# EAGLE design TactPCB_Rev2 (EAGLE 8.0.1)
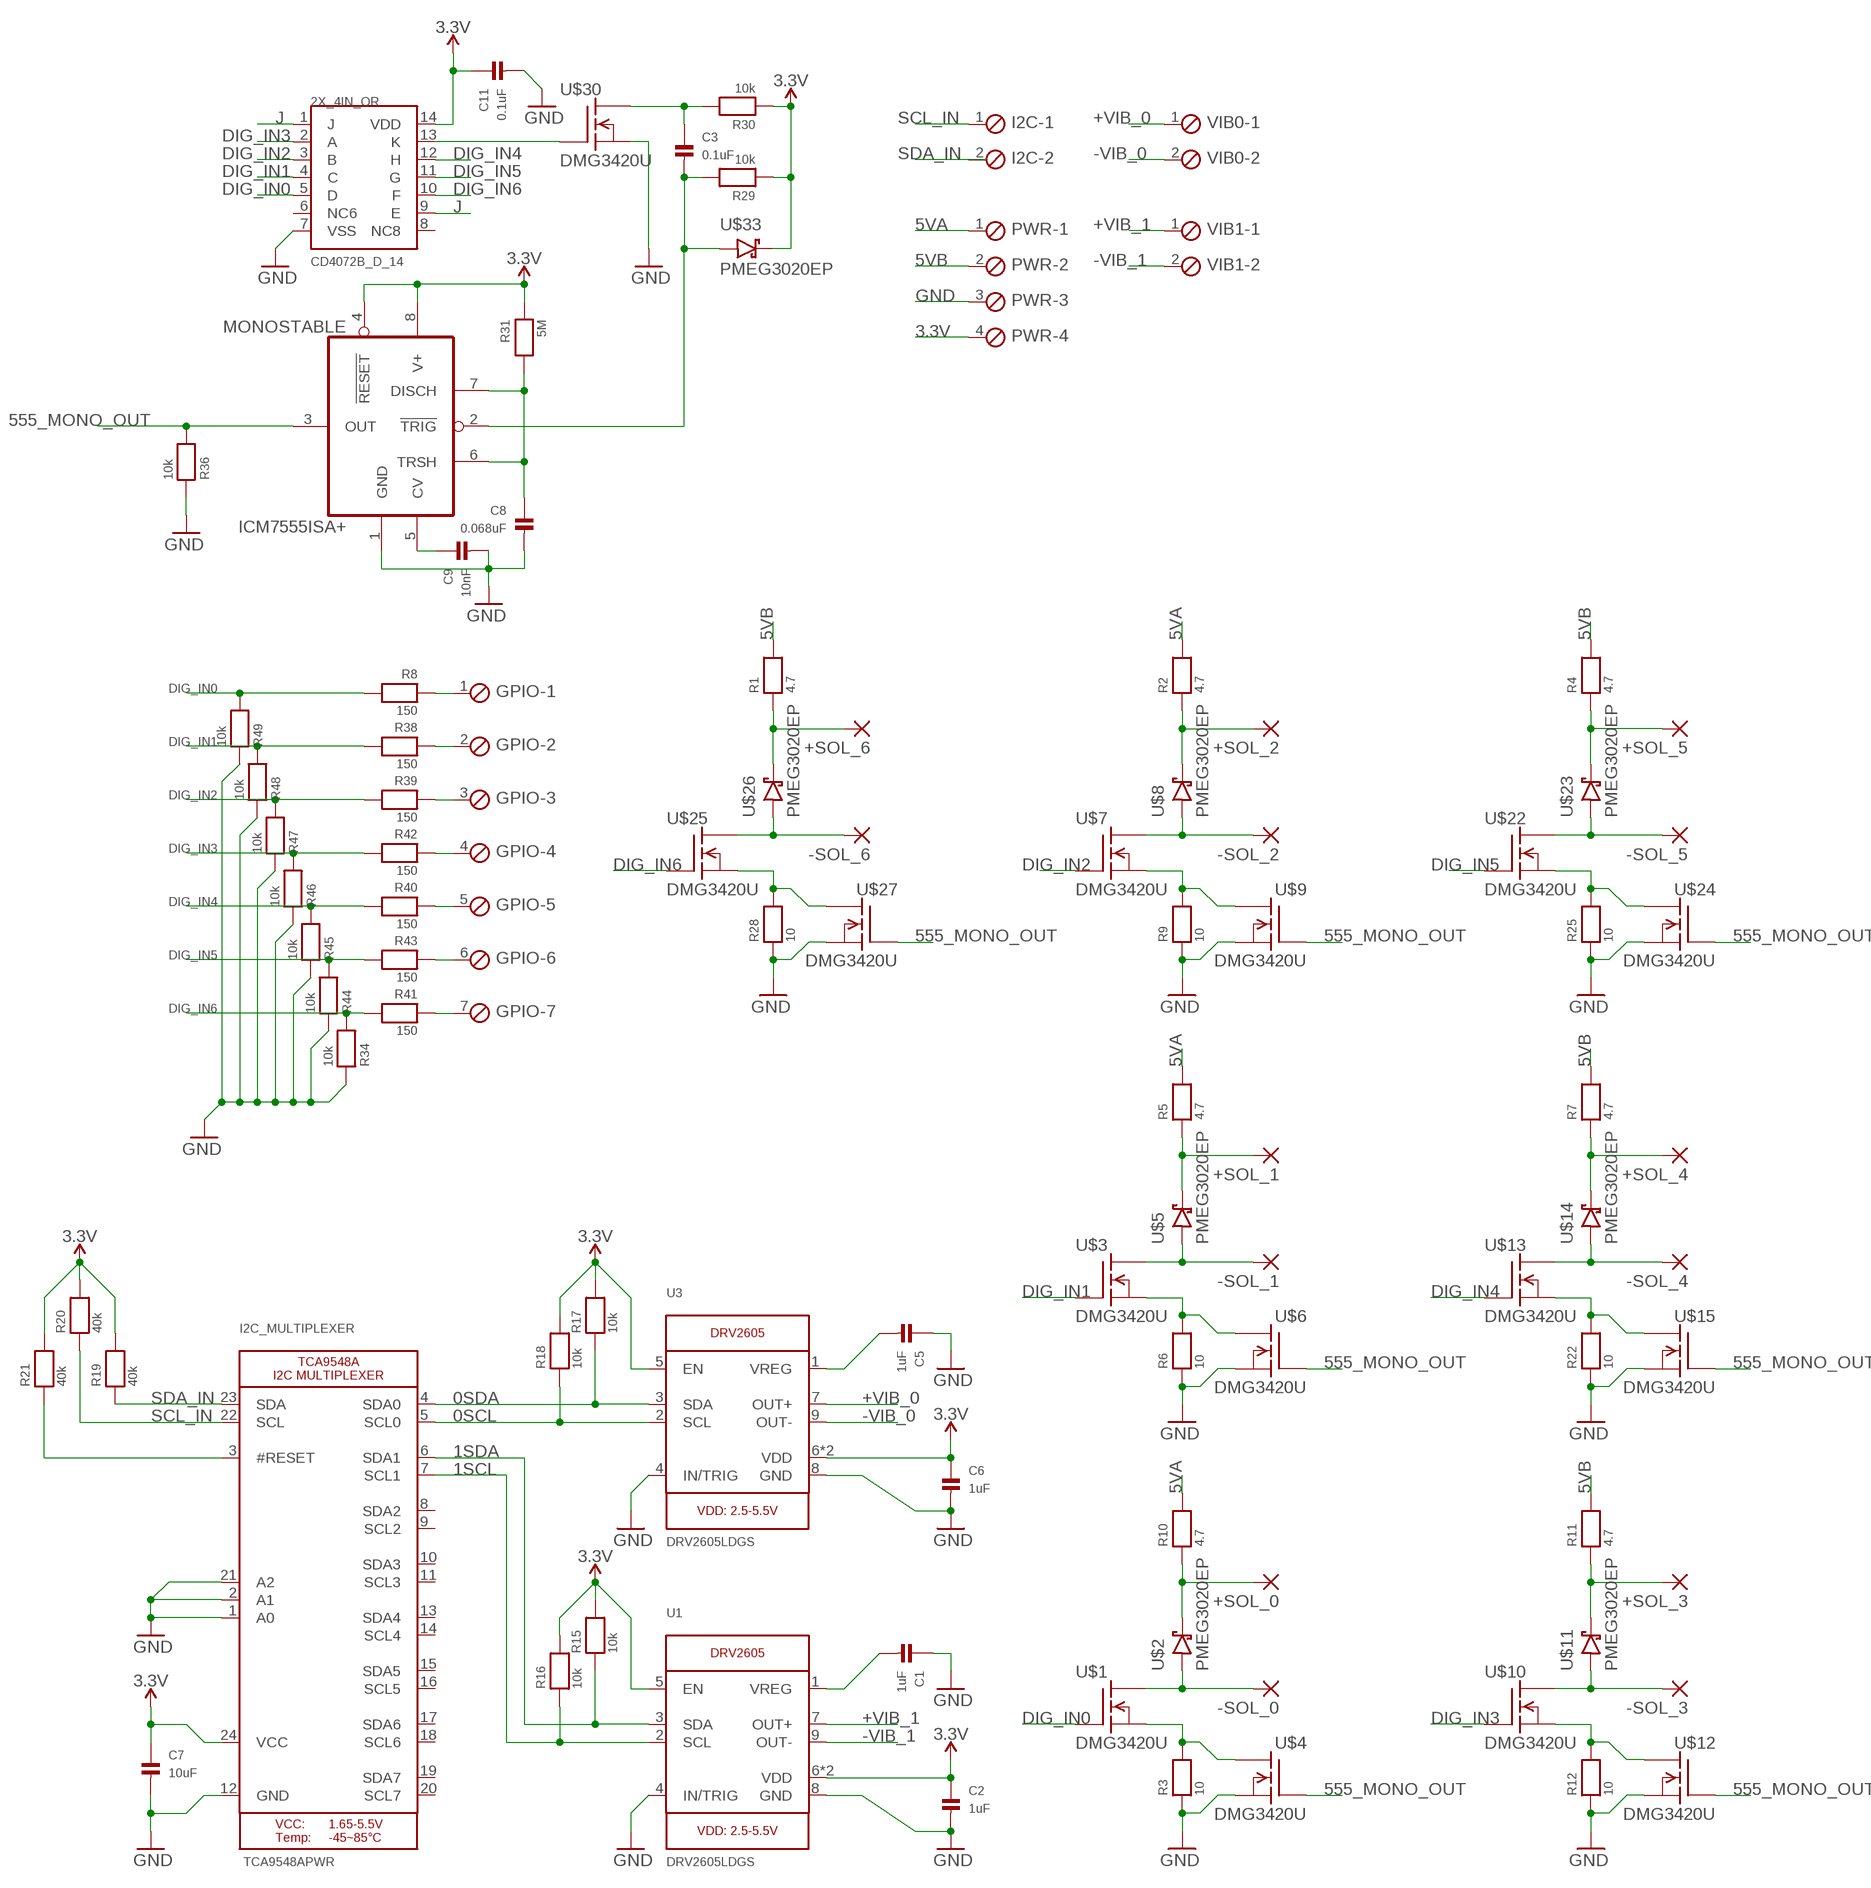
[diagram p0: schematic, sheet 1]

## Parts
2X_4IN_OR  CD4072B_D_14  [SOIC-14]
+SOL_0  2,15/1,0  [2,15/1,0]
+SOL_1  2,15/1,0  [2,15/1,0]
+SOL_2  2,15/1,0  [2,15/1,0]
+SOL_3  2,15/1,0  [2,15/1,0]
+SOL_4  2,15/1,0  [2,15/1,0]
+SOL_5  2,15/1,0  [2,15/1,0]
+SOL_6  2,15/1,0  [2,15/1,0]
-SOL_0  2,15/1,0  [2,15/1,0]
-SOL_1  2,15/1,0  [2,15/1,0]
-SOL_2  2,15/1,0  [2,15/1,0]
-SOL_3  2,15/1,0  [2,15/1,0]
-SOL_4  2,15/1,0  [2,15/1,0]
-SOL_5  2,15/1,0  [2,15/1,0]
-SOL_6  2,15/1,0  [2,15/1,0]
C1  1uF  CAP_CERAMIC0805  [0805]
C2  1uF  CAP_CERAMIC0805  [0805]
C3  0.1uF  CAP_CERAMIC0805  [0805]
C5  1uF  CAP_CERAMIC0805  [0805]
C6  1uF  CAP_CERAMIC0805  [0805]
C7  10uF  CAP_CERAMIC0805  [0805]
C8  0.068uF  CAP_CERAMIC0805  [0805]
C9  10nF  CAP_CERAMIC0805  [0805]
C11  0.1uF  CAP_CERAMIC0805  [0805]
GPIO  MPT7  [7POL254]
I2C  MPT2  [2POL254]
I2C_MULTIPLEXER  TCA9548APWR  TCA9548A  [TSSOP24]
MONOSTABLE  ICM7555ISA+  [SOIC-8]
PWR  MPT4  [4POL254]
R1  4.7  RESISTOR0805  [0805]
R2  4.7  RESISTOR0805  [0805]
R3  10  RESISTOR0805  [0805]
R4  4.7  RESISTOR0805  [0805]
R5  4.7  RESISTOR0805  [0805]
R6  10  RESISTOR0805  [0805]
R7  4.7  RESISTOR0805  [0805]
R8  150  RESISTOR0805  [0805]
R9  10  RESISTOR0805  [0805]
R10  4.7  RESISTOR0805  [0805]
R11  4.7  RESISTOR0805  [0805]
R12  10  RESISTOR0805  [0805]
R15  10k  RESISTOR0805  [0805]
R16  10k  RESISTOR0805  [0805]
R17  10k  RESISTOR0805  [0805]
R18  10k  RESISTOR0805  [0805]
R19  40k  RESISTOR0805  [0805]
R20  40k  RESISTOR0805  [0805]
R21  40k  RESISTOR0805  [0805]
R22  10  RESISTOR0805  [0805]
R25  10  RESISTOR0805  [0805]
R28  10  RESISTOR0805  [0805]
R29  10k  RESISTOR0805  [0805]
R30  10k  RESISTOR0805  [0805]
R31  5M  RESISTOR0805  [0805]
R34  10k  RESISTOR0805  [0805]
R36  10k  RESISTOR0805  [0805]
R38  150  RESISTOR0805  [0805]
R39  150  RESISTOR0805  [0805]
R40  150  RESISTOR0805  [0805]
R41  150  RESISTOR0805  [0805]
R42  150  RESISTOR0805  [0805]
R43  150  RESISTOR0805  [0805]
R44  10k  RESISTOR0805  [0805]
R45  10k  RESISTOR0805  [0805]
R46  10k  RESISTOR0805  [0805]
R47  10k  RESISTOR0805  [0805]
R48  10k  RESISTOR0805  [0805]
R49  10k  RESISTOR0805  [0805]
U1  DRV2605LDGS  DRV2605_SOP  [PSOP10]
U3  DRV2605LDGS  DRV2605_SOP  [PSOP10]
U$1  DMG3420U  [SOT23-3]
U$2  PMEG3020EP  [SOD128]
U$3  DMG3420U  [SOT23-3]
U$4  DMG3420U  [SOT23-3]
U$5  PMEG3020EP  [SOD128]
U$6  DMG3420U  [SOT23-3]
U$7  DMG3420U  [SOT23-3]
U$8  PMEG3020EP  [SOD128]
U$9  DMG3420U  [SOT23-3]
U$10  DMG3420U  [SOT23-3]
U$11  PMEG3020EP  [SOD128]
U$12  DMG3420U  [SOT23-3]
U$13  DMG3420U  [SOT23-3]
U$14  PMEG3020EP  [SOD128]
U$15  DMG3420U  [SOT23-3]
U$22  DMG3420U  [SOT23-3]
U$23  PMEG3020EP  [SOD128]
U$24  DMG3420U  [SOT23-3]
U$25  DMG3420U  [SOT23-3]
U$26  PMEG3020EP  [SOD128]
U$27  DMG3420U  [SOT23-3]
U$30  DMG3420U  [SOT23-3]
U$33  PMEG3020EP  [SOD128]
VIB0  MPT2  [2POL254]
VIB1  MPT2  [2POL254]

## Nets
0SCL: I2C_MULTIPLEXER.5(SCL0) R18.1 U3.2(SCL)
0SDA: I2C_MULTIPLEXER.4(SDA0) R17.1 U3.3(SDA)
1SCL: I2C_MULTIPLEXER.7(SCL1) R16.1 U1.2(SCL)
1SDA: I2C_MULTIPLEXER.6(SDA1) R15.1 U1.3(SDA)
3.3V: 2X_4IN_OR.14(VDD) C2.1 C6.1 C7.1 C11.1 I2C_MULTIPLEXER.24(VCC) MONOSTABLE.4(!RESET) MONOSTABLE.8(V+) PWR.4 R15.2 R16.2 R17.2 R18.2 R19.2 R20.2 R21.2 R29.1 R30.1 R31.1 U1.5(EN) U1.6(VDD) U1.10(VDD) U3.5(EN) U3.6(VDD) U3.10(VDD) U$33.2
5VA: PWR.1 R2.2 R5.2 R10.2
5VB: PWR.2 R1.2 R4.2 R7.2 R11.2
555_MONO_OUT: MONOSTABLE.3(OUT) R36.2 U$4.1(G) U$6.1(G) U$9.1(G) U$12.1(G) U$15.1(G) U$24.1(G) U$27.1(G)
+VIB_0: U3.7(OUT+) VIB0.1
+VIB_1: U1.7(OUT+) VIB1.1
-VIB_0: U3.9(OUT-) VIB0.2
-VIB_1: U1.9(OUT-) VIB1.2
DIG_IN0: 2X_4IN_OR.5(D) R8.2 R49.2 U$1.1(G)
DIG_IN1: 2X_4IN_OR.4(C) R38.2 R48.2 U$3.1(G)
DIG_IN2: 2X_4IN_OR.3(B) R39.2 R47.2 U$7.1(G)
DIG_IN3: 2X_4IN_OR.2(A) R42.2 R46.2 U$10.1(G)
DIG_IN4: 2X_4IN_OR.12(H) R40.2 R45.2 U$13.1(G)
DIG_IN5: 2X_4IN_OR.11(G) R43.2 R44.2 U$22.1(G)
DIG_IN6: 2X_4IN_OR.10(F) R34.2 R41.2 U$25.1(G)
GND: 2X_4IN_OR.7(VSS) C1.1 C2.2 C5.1 C6.2 C7.2 C8.2 C9.2 C11.2 I2C_MULTIPLEXER.1(A0) I2C_MULTIPLEXER.2(A1) I2C_MULTIPLEXER.12(GND) I2C_MULTIPLEXER.21(A2) MONOSTABLE.1(GND) PWR.3 R3.1 R6.1 R9.1 R12.1 R22.1 R25.1 R28.1 R34.1 R36.1 R44.1 R45.1 R46.1 R47.1 R48.1 R49.1 U1.4(IN/TRIG) U1.8(GND) U3.4(IN/TRIG) U3.8(GND) U$4.3(S) U$6.3(S) U$9.3(S) U$12.3(S) U$15.3(S) U$24.3(S) U$27.3(S) U$30.3(S)
J: 2X_4IN_OR.1(J) 2X_4IN_OR.9(E)
N$1: R3.2 U$1.3(S) U$4.2(D)
N$2: +SOL_6.1(P) R1.1 U$26.2
N$3: -SOL_0.1(P) U$1.2(D) U$2.1
N$4: +SOL_2.1(P) R2.1 U$8.2
N$5: -SOL_1.1(P) U$3.2(D) U$5.1
N$6: R6.2 U$3.3(S) U$6.2(D)
N$7: +SOL_5.1(P) R4.1 U$23.2
N$8: -SOL_2.1(P) U$7.2(D) U$8.1
N$9: R9.2 U$7.3(S) U$9.2(D)
N$10: +SOL_4.1(P) R7.1 U$14.2
N$11: -SOL_3.1(P) U$10.2(D) U$11.1
N$12: R12.2 U$10.3(S) U$12.2(D)
N$13: +SOL_1.1(P) R5.1 U$5.2
N$14: -SOL_4.1(P) U$13.2(D) U$14.1
N$15: C1.2 U1.1(VREG)
N$16: C5.2 U3.1(VREG)
N$17: C3.1 R30.2 U$30.2(D)
N$18: C3.2 MONOSTABLE.2(!TRIG) R29.2 U$33.1
N$19: +SOL_0.1(P) R10.1 U$2.2
N$20: +SOL_3.1(P) R11.1 U$11.2
N$23: R22.2 U$13.3(S) U$15.2(D)
N$25: -SOL_5.1(P) U$22.2(D) U$23.1
N$26: R25.2 U$22.3(S) U$24.2(D)
N$28: -SOL_6.1(P) U$25.2(D) U$26.1
N$29: R28.2 U$25.3(S) U$27.2(D)
N$32: C9.1 MONOSTABLE.5(CV)
N$33: C8.1 MONOSTABLE.6(TRSH) MONOSTABLE.7(DISCH) R31.2
N$34: 2X_4IN_OR.13(K) U$30.1(G)
N$41: GPIO.1 R8.1
N$46: GPIO.7 R41.1
N$47: GPIO.3 R39.1
N$48: GPIO.5 R40.1
N$111: GPIO.2 R38.1
N$112: GPIO.4 R42.1
N$113: GPIO.6 R43.1
RESET: I2C_MULTIPLEXER.3(#RESET) R21.1
SCL_IN: I2C.1 I2C_MULTIPLEXER.22(SCL) R20.1
SDA_IN: I2C.2 I2C_MULTIPLEXER.23(SDA) R19.1
Unconnected: 2X_4IN_OR.6(NC6) 2X_4IN_OR.8(NC8) I2C_MULTIPLEXER.8(SDA2) I2C_MULTIPLEXER.9(SCL2) I2C_MULTIPLEXER.10(SDA3) I2C_MULTIPLEXER.11(SCL3) I2C_MULTIPLEXER.13(SDA4) I2C_MULTIPLEXER.14(SCL4) I2C_MULTIPLEXER.15(SDA5) I2C_MULTIPLEXER.16(SCL5) I2C_MULTIPLEXER.17(SDA6) I2C_MULTIPLEXER.18(SCL6) I2C_MULTIPLEXER.19(SDA7) I2C_MULTIPLEXER.20(SCL7)

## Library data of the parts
2X_4IN_OR = SD2017_StephenMiles:CD4072B_D_14
+SOL_0 +SOL_1-+SOL_6 -SOL_0 -SOL_1--SOL_6 = wirepad:2,15/1,0: THROUGH-HOLE PAD
C1-C3 C5-C9 C11 = microbuilder:CAP_CERAMIC: Ceramic Capacitors
GPIO = con-phoenix-254:MPT7: PHOENIX CONNECTOR; OC_FARNELL: unknown; OC_NEWARK: unknown
I2C VIB0 VIB1 = con-phoenix-254:MPT2: PHOENIX CONNECTOR; OC_FARNELL: unknown; OC_NEWARK: unknown
I2C_MULTIPLEXER = TactilePCB:TCA9548A: TCA9548A I2C Multiplexer
MONOSTABLE = SD2017_StephenMiles:ICM7555ISA+
PWR = con-phoenix-254:MPT4: PHOENIX CONNECTOR; OC_FARNELL: unknown; OC_NEWARK: unknown
R1-R12 R15-R22 R25 R28-R31 R34 R36 R38-R49 = microbuilder:RESISTOR: Resistors
U1 U3 = TactilePCB:DRV2605: DRV2605 - Haptic Driver for ERM/LRA Motors
U$1 U$3 U$4 U$6 U$7 U$9 U$10 U$12 U$13 U$15 U$22 U$24 U$25 U$27 U$30 = SD2017_StephenMiles:DMG3420U: N-Channel MosFET 20Vds, 1Vgs(th), 5.47A Id
U$2 U$5 U$8 U$11 U$14 U$23 U$26 U$33 = SD2017_StephenMiles:PMEG3020EP: Schottky Diode

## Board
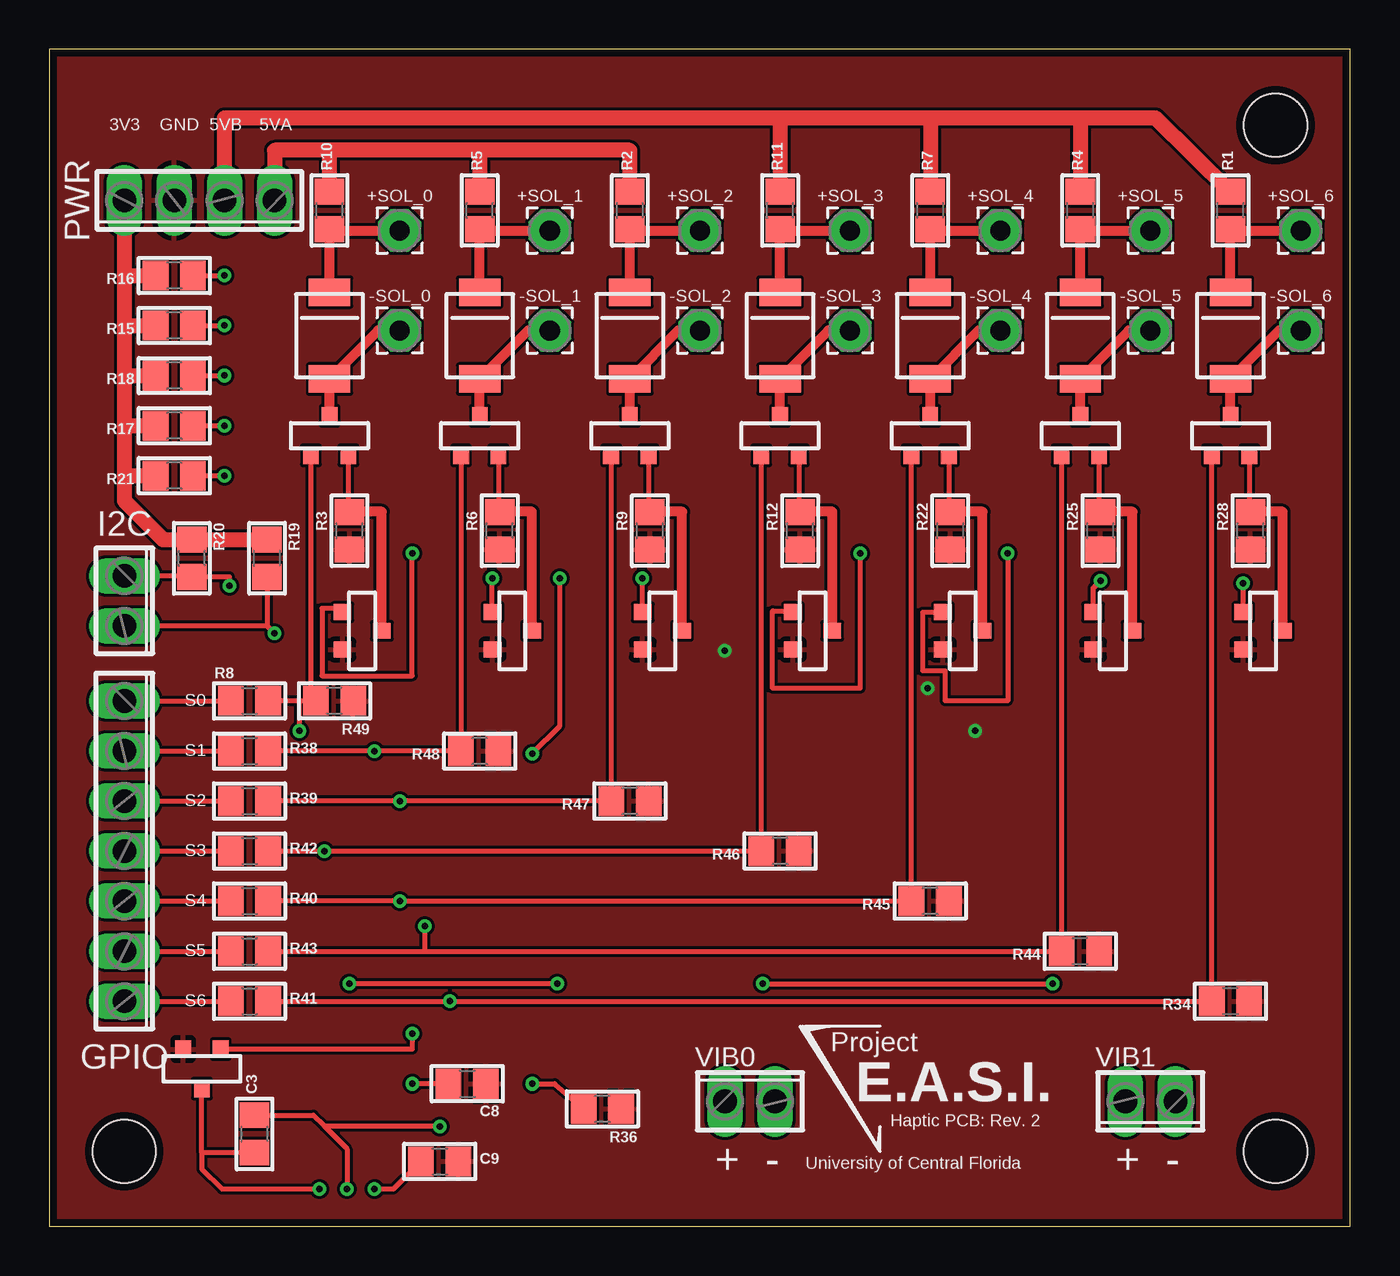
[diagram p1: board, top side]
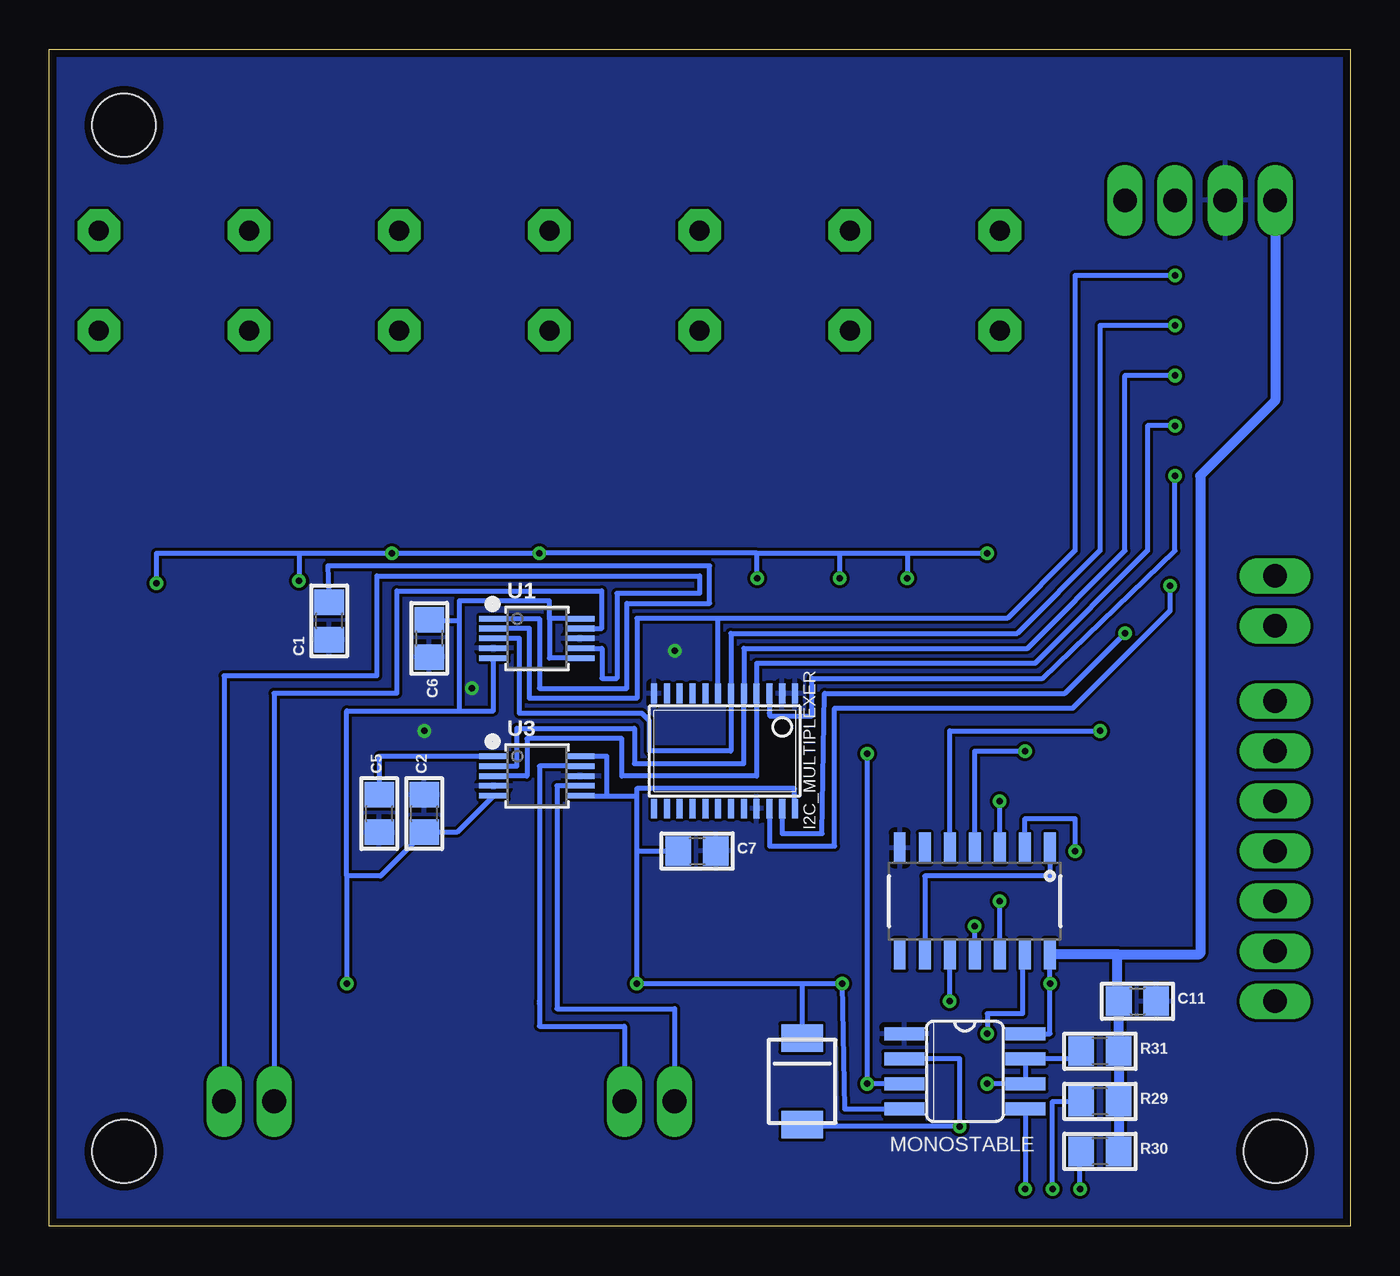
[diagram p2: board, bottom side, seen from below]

Size 66.02 x 59.74 mm. Coordinates in mm from the lower left corner, seen from the top.
Outline: 0,0 66.02,0 66.02,59.74 0,59.74 0,0
Copper layers (1*16): Top 0.0356mm / dielectric 1.5011mm / Bottom 0.0356mm
Design rules "oshpark-2layer": minimum track width 6mil, minimum drill 13mil, track to track 6mil, track to pad 6mil, pad to pad 6mil, via to via 6mil, smd to smd 6mil, copper to edge 15mil, drill to drill 6mil, minimum pad ring 7mil, minimum via ring 7mil, stop-mask expansion 2.5mil, vias tented up to drill 0mil, thermal gap 10mil
Holes 3.2 mm at 62.23,3.81 3.81,3.81 62.23,55.88

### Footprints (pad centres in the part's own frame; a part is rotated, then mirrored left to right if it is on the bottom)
SOIC-14 = smd 0.6 x 1.55: 1 -3.81,-2.7; 2 -2.54,-2.7; 3 -1.27,-2.7; 4 0,-2.7; 5 1.27,-2.7; 6 2.54,-2.7; 7 3.81,-2.7; 8 3.81,2.7; 9 2.54,2.7; 10 1.27,2.7; 11 0,2.7; 12 -1.27,2.7; 13 -2.54,2.7; 14 -3.81,2.7
2,15/1,0 = drill 1.016 pad 2.159 octagon: 1 0,0
0805 = smd 1.3 x 1.5: 1 -0.95,0; 2 0.95,0
7POL254 = drill 1.2 long: 1 -7.62,0; 2 -5.08,0; 3 -2.54,0; 4 0,0; 5 2.54,0; 6 5.08,0; 7 7.62,0
2POL254 = drill 1.2 long: 1 -1.27,0; 2 1.27,0
TSSOP24 = smd 0.305 x 0.991: 1 -3.575,-2.918; 2 -2.925,-2.918; 3 -2.275,-2.918; 4 -1.625,-2.918; 5 -0.975,-2.918; 6 -0.325,-2.918; 7 0.325,-2.918; 8 0.975,-2.918; 9 1.625,-2.918; 10 2.275,-2.918; 11 2.925,-2.918; 12 3.575,-2.918; 13 3.575,2.918; 14 2.925,2.918; 15 2.275,2.918; 16 1.625,2.918; 17 0.975,2.918; 18 0.325,2.918; 19 -0.325,2.918; 20 -0.975,2.918; 21 -1.625,2.918; 22 -2.275,2.918; 23 -2.925,2.918; 24 -3.575,2.918
SOIC-8 = smd 0.66 x 2.032: 1 -1.905,-3.073; 2 -0.635,-3.073; 3 0.635,-3.073; 4 1.905,-3.073; 5 1.905,3.073; 6 0.635,3.073; 7 -0.635,3.073; 8 -1.905,3.073
4POL254 = drill 1.2 long: 1 -3.81,0; 2 -1.27,0; 3 1.27,0; 4 3.81,0
PSOP10 = smd 0.28 x 1.45: 1 -1,-2.2; 2 -0.5,-2.2; 3 0,-2.2; 4 0.5,-2.2; 5 1,-2.2; 6 1,2.2; 7 0.5,2.2; 8 0,2.2; 9 -0.5,2.2; 10 -1,2.2
SOT23-3 = smd 0.8 x 0.9: 1 -0.95,-1; 2 0,1; 3 0.95,-1
SOD128 = smd 1.4 x 2.1: 1 -2.2,0; 2 2.2,0

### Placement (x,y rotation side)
2X_4IN_OR  19.05,16.51 180 bottom
+SOL_0  17.78,50.55 0 top
+SOL_1  25.4,50.55 0 top
+SOL_2  33.02,50.55 0 top
+SOL_3  40.64,50.55 0 top
+SOL_4  48.26,50.55 0 top
+SOL_5  55.88,50.55 0 top
+SOL_6  63.5,50.55 0 top
-SOL_0  17.78,45.47 0 top
-SOL_1  25.4,45.47 0 top
-SOL_2  33.02,45.47 0 top
-SOL_3  40.64,45.47 0 top
-SOL_4  48.26,45.47 0 top
-SOL_5  55.88,45.47 0 top
-SOL_6  63.5,45.47 0 top
C1  51.82,30.73 90 bottom
C2  46.99,20.95 90 bottom
C3  10.41,4.7 90 top
C5  49.28,20.95 90 bottom
C6  46.74,29.84 270 bottom
C7  33.15,19.05 0 bottom
C8  21.21,7.24 0 top
C9  19.81,3.3 0 top
C11  10.79,11.43 0 bottom
GPIO  3.81,19.05 270 top
I2C  3.81,31.75 270 top
I2C_MULTIPLEXER  31.75,24.13 180 bottom
MONOSTABLE  19.56,7.87 270 bottom
PWR  7.62,52.07 180 top
R1  59.94,51.56 90 top
R2  29.46,51.56 90 top
R3  15.24,35.31 90 top
R4  52.32,51.56 90 top
R5  21.84,51.56 90 top
R6  22.86,35.31 90 top
R7  44.7,51.56 90 top
R8  10.16,26.67 0 top
R9  30.48,35.31 90 top
R10  14.22,51.56 90 top
R11  37.08,51.56 90 top
R12  38.1,35.31 90 top
R15  6.35,45.72 180 top
R16  6.35,48.26 180 top
R17  6.35,40.64 180 top
R18  6.35,43.18 180 top
R19  11.05,33.91 90 top
R20  7.24,33.91 90 top
R21  6.35,38.1 180 top
R22  45.72,35.31 90 top
R25  53.34,35.31 90 top
R28  60.96,35.31 90 top
R29  12.7,6.35 180 bottom
R30  12.7,3.81 180 bottom
R31  12.7,8.89 180 bottom
R34  59.94,11.43 180 top
R36  28.07,5.97 180 top
R38  10.16,24.13 0 top
R39  10.16,21.59 0 top
R40  10.16,16.51 0 top
R41  10.16,11.43 0 top
R42  10.16,19.05 0 top
R43  10.16,13.97 0 top
R44  52.32,13.97 180 top
R45  44.7,16.51 180 top
R46  37.08,19.05 180 top
R47  29.46,21.59 180 top
R48  21.84,24.13 180 top
R49  14.48,26.67 180 top
U1  41.27,29.84 270 bottom
U3  41.27,22.86 270 bottom
U$1  14.22,40.13 0 top
U$2  14.22,45.21 90 top
U$3  21.84,40.13 0 top
U$4  15.88,30.23 270 top
U$5  21.84,45.21 90 top
U$6  23.5,30.23 270 top
U$7  29.46,40.13 0 top
U$8  29.46,45.21 90 top
U$9  31.11,30.23 270 top
U$10  37.08,40.13 0 top
U$11  37.08,45.21 90 top
U$12  38.73,30.23 270 top
U$13  44.7,40.13 0 top
U$14  44.7,45.21 90 top
U$15  46.35,30.23 270 top
U$22  52.32,40.13 0 top
U$23  52.32,45.21 90 top
U$24  53.98,30.23 270 top
U$25  59.94,40.13 0 top
U$26  59.94,45.21 90 top
U$27  61.59,30.23 270 top
U$30  7.75,8 180 top
U$33  27.81,7.37 90 bottom
VIB0  35.56,6.35 0 top
VIB1  55.88,6.35 180 top

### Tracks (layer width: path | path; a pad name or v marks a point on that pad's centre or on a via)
0SCL  (via drill 0.33 pad 0.13)
  Top 0.254: R18.1 v8.89,43.18
  Bottom 0.254: v8.89,43.18 11.43,43.18 11.43,34.29 16.38,29.34 30.77,29.34 I2C_MULTIPLEXER.5 30.77,23.5 36.32,23.5 36.32,25.27 42.29,25.27 42.29,23.37 U3.2
0SDA  (via drill 0.33 pad 0.13)
  Top 0.254: R17.1 v8.89,40.64
  Bottom 0.254: v8.89,40.64 10.29,40.64 10.29,34.29 16,28.57 30.12,28.57 I2C_MULTIPLEXER.4 30.12,22.86 36.96,22.86 36.96,24.77 41.78,24.77 41.78,22.86 U3.3
1SCL  (via drill 0.33 pad 0.13)
  Top 0.254: R16.1 v8.89,48.26
  Bottom 0.254: v8.89,48.26 13.97,48.26 13.97,34.29 17.4,30.86 32.08,30.86 | I2C_MULTIPLEXER.7 32.08,30.86 | 32.08,30.86 36.2,30.86 36.2,26.8 41.66,26.8 41.66,30.35 43.48,30.35 U1.2
1SDA  (via drill 0.33 pad 0.13)
  Top 0.254: R15.1 v8.89,45.72
  Bottom 0.254: v8.89,45.72 12.7,45.72 12.7,34.29 16.89,30.1 31.43,30.1 I2C_MULTIPLEXER.6 31.43,24.13 35.56,24.13 35.56,25.65 35.94,26.04 42.16,26.04 42.16,29.84 U1.3
3.3V  (via drill 0.33 pad 0.13)
  Top 0.254: v25.78,12.32 v15.24,12.32 | v36.2,12.32 v50.93,12.32
  Top 0.762: 3.81,48.26 3.81,45.72 | 3.81,45.72 3.81,43.18 | 3.81,43.18 3.81,40.64 | 3.81,40.64 3.81,38.1 | 3.81,38.1 3.81,36.83 5.78,34.86 R20.2 R19.2 | 3.81,38.1 R21.2 | 3.81,40.64 R17.2 | 3.81,43.18 R18.2 | 3.81,45.72 R15.2 | 3.81,48.26 R16.2 | PWR.4 3.81,48.26
  Bottom 0.254: MONOSTABLE.4 25.65,5.97 v25.78,12.32 27.81,12.32 | R31.1 | 27.81,12.32 U$33.2 | I2C_MULTIPLEXER.24 28.19,21.21 28.19,22.23 36.2,22.23 36.2,21.84 | 36.2,19.05 36.2,21.84 | 36.2,19.05 C7.1 | U3.6 39.08,21.84 37.72,21.84 | 37.72,21.84 36.2,21.84 | 37.72,21.84 37.72,23.86 U3.10 | U1.6 40.64,28.84 40.64,30.84 | 40.64,30.84 40.64,31.75 45.21,31.75 45.21,30.73 | 39.08,30.86 U1.10 40.64,30.84 | 45.21,30.73 45.97,30.73 C6.1 | 27.81,12.32 v36.2,12.32 36.2,19.05 | MONOSTABLE.8 15.24,9.78 v15.24,12.32 2X_4IN_OR.14 | 45.21,30.73 45.21,26.16 | 45.21,26.16 50.93,26.16 50.93,17.78 | 43.56,28.76 U1.5 43.48,26.16 45.21,26.16 | 50.93,17.78 v50.93,12.32 50.8,12.32 | U3.5 45.33,20 C2.1 49.22,17.78 50.93,17.78
  Bottom 0.508: 15.21,13.84 2X_4IN_OR.14 11.81,13.81 | 11.81,13.81 7.65,13.81 7.62,13.84 7.62,38.1 3.81,41.91 PWR.4 | R31.1 C11.1 11.81,11.43 11.81,13.81 | R31.1 R29.1 R30.1
5VA
  Top 0.762: R10.2 14.22,54.61 | 21.84,54.61 14.22,54.61 | 21.84,54.61 R5.2 | R2.2 29.46,54.61 21.84,54.61 | 14.22,54.61 11.43,54.61 PWR.1
5VB
  Top 0.762: PWR.2 8.89,56.26 37.08,56.26 | 37.08,56.26 R11.2 | 37.08,56.26 44.7,56.26 | 44.7,56.26 R7.2 | 44.7,56.26 52.32,56.26 | 52.32,56.26 R4.2 | 52.32,56.26 56.13,56.26 R1.2
555_MONO_OUT  (via drill 0.33 pad 0.13)
  Top 0.254: v24.51,7.24 25.65,7.24 R36.2 | U$4.1 15.07,31.37 13.84,31.37 13.84,27.94 18.41,27.94 v18.41,34.16 | v24.51,24 25.91,25.4 v25.91,32.89 | U$6.1 22.48,31.18 v22.48,32.89 | U$9.1 v30.1,32.89 | v41.15,34.16 41.15,27.3 36.7,27.3 36.7,31.24 37.73,31.24 U$12.1 | U$24.1 52.98,32.4 v53.34,32.77 | v48.64,34.16 48.64,26.67 45.47,26.67 45.47,28.19 44.32,28.19 44.32,31.18 U$15.1 | U$27.1 60.59,32.64 v60.58,32.64
  Bottom 0.254: MONOSTABLE.3 v24.51,7.24 v24.51,24 | 30.1,34.16 v41.15,34.16 v48.64,34.16 53.34,34.16 | 30.1,34.16 25.91,34.16 | v60.58,32.64 60.58,34.16 53.34,34.16 | 53.34,34.16 v53.34,32.77 | v25.91,32.89 25.91,34.16 | 22.48,34.16 v18.41,34.16 | 22.48,34.16 v22.48,32.89 | 25.91,34.16 22.48,34.16 | v30.1,32.89 30.1,34.16
+VIB_0
  Bottom 0.254: U3.7 40.26,22.36 40.26,11.05 34.29,11.05 VIB0.1
+VIB_1
  Bottom 0.254: U1.7 37.97,29.34 37.97,27.81 37.21,27.81 37.21,32.13 33.02,32.13 33.02,33.02 49.4,33.02 49.4,27.94 57.15,27.94 VIB1.1
-VIB_0
  Bottom 0.254: U3.9 41.15,23.36 41.15,11.43 | 41.15,11.43 41.15,11.3 | 41.15,11.43 41.15,10.16 36.83,10.16 VIB0.2
-VIB_1
  Bottom 0.254: U1.9 39.08,30.35 37.97,30.35 37.97,32.26 48.39,32.26 48.39,27.05 54.61,27.05 VIB1.2
DIG_IN0  (via drill 0.33 pad 0.13)
  Top 0.254: 12.7,26.67 R8.2 | 12.7,26.67 R49.2 13.27,26.67 U$1.1 | v12.7,25.15 12.7,26.67
  Bottom 0.254: v12.7,25.15 20.32,25.15 2X_4IN_OR.5
DIG_IN1  (via drill 0.33 pad 0.13)
  Top 0.254: R38.2 v16.51,24.13 R48.2 U$3.1
  Bottom 0.254: 2X_4IN_OR.4 19.05,24.13 v16.51,24.13
DIG_IN2  (via drill 0.33 pad 0.13)
  Top 0.254: R39.2 v17.78,21.59 R47.2 U$7.1
  Bottom 0.254: 2X_4IN_OR.3 v17.78,21.59
DIG_IN3  (via drill 0.33 pad 0.13)
  Top 0.254: R42.2 v13.97,19.05 R46.2 U$10.1
  Bottom 0.254: 2X_4IN_OR.2 | 2X_4IN_OR.2 16.51,20.7 13.97,20.7 v13.97,19.05
DIG_IN4  (via drill 0.33 pad 0.13)
  Top 0.254: R40.2 v17.78,16.51 R45.2 U$13.1
  Bottom 0.254: 2X_4IN_OR.12 v17.78,16.51
DIG_IN5  (via drill 0.33 pad 0.13)
  Top 0.254: R43.2 19.05,13.97 | v19.05,15.24 19.05,13.97 | 19.05,13.97 R44.2 U$22.1
  Bottom 0.254: 2X_4IN_OR.11 v19.05,15.24
DIG_IN6  (via drill 0.33 pad 0.13)
  Top 0.254: R41.2 v20.32,11.43 R34.2 U$25.1
  Bottom 0.254: v20.32,11.43 2X_4IN_OR.10
GND  (via drill 0.33 pad 0.13)
  other vias: 34.29,29.21 46.99,25.15 44.58,27.3
  pour Top: 0,59.69 0,0 66.04,0 66.04,59.69
  pour Bottom: 0,59.69 0,0 66.04,0 66.04,59.69
J
  Bottom 0.254: 2X_4IN_OR.1 15.24,17.78 21.59,17.78 2X_4IN_OR.9
N$1
  Top 0.254: U$1.3 15.17,36.32 R3.2
  Top 0.508: U$4.2 16.88,36.27 15.24,36.27 R3.2
N$2
  Top 0.508: U$26.2 R1.1 60.01,50.55 +SOL_6.1
N$3
  Top 0.508: U$1.2 U$2.1 16.68,45.47 -SOL_0.1
N$4
  Top 0.508: U$8.2 R2.1 29.53,50.55 +SOL_2.1
N$5
  Top 0.508: U$3.2 U$5.1 24.3,45.47 -SOL_1.1
N$6
  Top 0.254: U$3.3 22.79,36.32 R6.2
  Top 0.508: U$6.2 24.5,36.27 22.86,36.27 R6.2
N$7
  Top 0.508: U$23.2 R4.1 52.39,50.55 +SOL_5.1
N$8
  Top 0.508: U$7.2 U$8.1 31.92,45.47 -SOL_2.1
N$9
  Top 0.254: U$7.3 30.41,36.32 R9.2
  Top 0.508: U$9.2 32.12,36.27 30.48,36.27 R9.2
N$10
  Top 0.508: U$14.2 R7.1 44.77,50.55 +SOL_4.1
N$11
  Top 0.508: U$10.2 U$11.1 39.54,45.47 -SOL_3.1
N$12
  Top 0.254: U$10.3 38.03,36.32 R12.2
  Top 0.508: U$12.2 39.73,36.27 38.1,36.27 R12.2
N$13
  Top 0.508: U$5.2 R5.1 21.91,50.55 +SOL_1.1
N$14
  Top 0.508: U$13.2 U$14.1 47.16,45.47 -SOL_4.1
N$15
  Bottom 0.254: U1.1 41.15,30.84 41.15,27.3 36.7,27.3 36.7,31.62 32.51,31.62 32.51,33.53 51.88,33.53 C1.2
N$16
  Bottom 0.254: U3.1 49.28,23.86 C5.2
N$17  (via drill 0.33 pad 0.13)
  Top 0.254: C3.1 7.75,3.75 | 7.75,3.75 U$30.2 | 7.75,3.75 7.75,2.92 8.76,1.91 v13.72,1.91
  Bottom 0.254: v13.72,1.91 13.72,3.74 R30.2
N$18  (via drill 0.33 pad 0.13)
  Top 0.254: v15.11,1.91 15.11,3.94 13.97,5.08 | C3.2 13.4,5.65 13.97,5.08 | v19.81,5.08 13.97,5.08
  Bottom 0.254: MONOSTABLE.2 19.81,8.51 v19.81,5.08 27.22,5.08 U$33.1 | 13.72,6.35 R29.2 15.11,6.35 v15.11,1.91
N$19
  Top 0.508: U$2.2 R10.1 14.29,50.55 +SOL_0.1
N$20
  Top 0.508: U$11.2 R11.1 37.15,50.55 +SOL_3.1
N$23
  Top 0.254: U$13.3 45.65,36.32 R22.2
  Top 0.508: U$15.2 47.35,36.27 45.72,36.27 R22.2
N$25
  Top 0.508: U$22.2 U$23.1 54.78,45.47 -SOL_5.1
N$26
  Top 0.254: U$22.3 53.27,36.32 R25.2
  Top 0.508: U$24.2 54.98,36.27 53.34,36.27 R25.2
N$28
  Top 0.508: U$25.2 U$26.1 62.4,45.47 -SOL_6.1
N$29
  Top 0.254: U$25.3 60.89,36.32 R28.2
  Top 0.508: U$27.2 62.59,36.27 60.96,36.27 R28.2
N$32  (via drill 0.33 pad 0.13)
  Top 0.254: v16.51,1.91 17.46,1.91 C9.1
  Bottom 0.254: MONOSTABLE.5 16.48,1.93 v16.51,1.91
N$33  (via drill 0.33 pad 0.13)
  Top 0.254: C8.1 v18.41,7.24
  Bottom 0.254: R31.2 14.03,8.51 MONOSTABLE.7 MONOSTABLE.6 v18.41,7.24
N$34  (via drill 0.33 pad 0.13)
  Top 0.254: v18.41,9.78 18.41,9 U$30.1
  Bottom 0.254: 2X_4IN_OR.13 16.64,13.81 16.64,10.79 18.41,10.79 v18.41,9.78
N$41
  Top 0.254: GPIO.1 R8.1
N$46
  Top 0.254: GPIO.7 R41.1
N$47
  Top 0.254: GPIO.3 R39.1
N$48
  Top 0.254: GPIO.5 R40.1
N$111
  Top 0.254: GPIO.2 R38.1
N$112
  Top 0.254: R42.1 8.89,19.05 GPIO.4
N$113
  Top 0.254: GPIO.6 R43.1
RESET  (via drill 0.33 pad 0.13)
  Top 0.254: R21.1 v8.89,38.1
  Bottom 0.254: v8.89,38.1 8.89,34.29 15.62,27.81 27.3,27.81 27.3,25.91 29.46,25.91 29.46,26.04 29.48,26.04 I2C_MULTIPLEXER.3
SCL_IN  (via drill 0.33 pad 0.13)
  Top 0.254: I2C.1 6.99,33.02 R20.1 9.14,32.96 v9.14,32.51
  Bottom 0.254: 29.46,21.2 I2C_MULTIPLEXER.22 29.46,21.21 29.46,19.3 26.16,19.3 26.16,26.29 14.1,26.29 9.14,31.24 v9.14,32.51
SDA_IN  (via drill 0.33 pad 0.13)
  Top 0.254: 11.05,30.48 I2C.2 | v11.43,30.1 11.05,30.48 | R19.1 11.05,30.48
  Bottom 0.254: I2C_MULTIPLEXER.23 28.83,19.94 26.8,19.94 26.67,27.05 14.48,27.05 v11.43,30.1

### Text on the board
tPlace: 3V3 | GND | 5VB | 5VA | S0 | S1 | S2 | S3 | S4 | S5 | S6 | Project | E.A.S.I. | Haptic PCB: Rev. 2 | + | - | University of Central Florida | + | -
